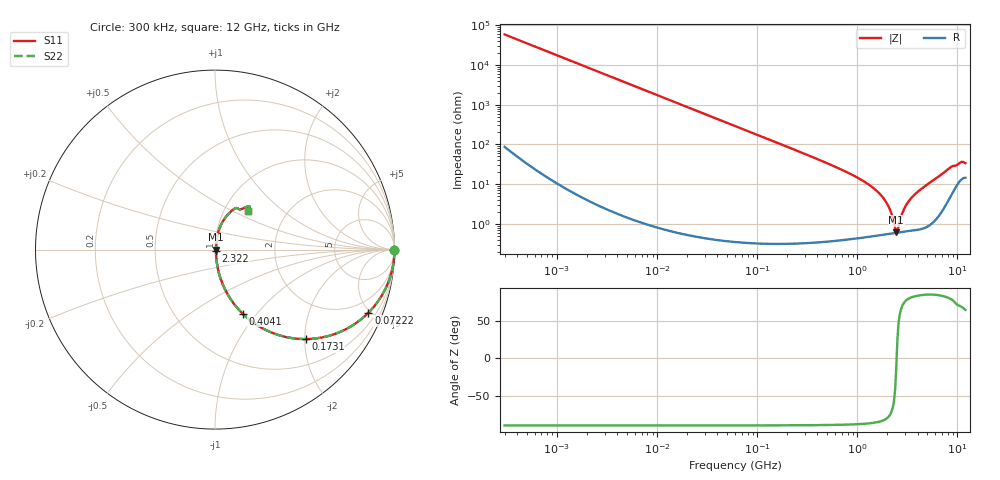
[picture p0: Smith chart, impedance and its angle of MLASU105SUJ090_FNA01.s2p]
! MLASU105SUJ090_FNA01  S-PARAMETER MODEL  ( General Type )
! Model Generated by TAIYO YUDEN Corporation (http://www.ty-top.com)
! Version 2.0
! TAIYO YUDEN Control No. 120810
! Copyright(c) 2012 TAIYO YUDEN CO.,LTD. All Rights Reserved.
! Product Description (link to TY-COMPAS)
! https://ds.yuden.co.jp/TYCOMPAS/or/detail?pn=MLASU105SUJ090DFNA01&u=M
! Products Name : Multilayer Ceramic Capacitors
! Characteristics :
!  Capacitance : 9 pF , Rated Voltage : 50V , TCC : UJ / U2J
!  Case Size : 1.0 x 0.5 / 0.039 x 0.02 [mm/inch] , Thickness : 0.5 / 0.02 [mm/inch]
!  (Conditions: Temperature = 25 degC , DC Bias Current/Voltage = 0A / 0V)
! External Node Assignments :
!  1  o---| |---o  2
! GND o---------o GND
! Frequency Range : 0.3MHz  -  12000MHz  [ 401 STEP ]
# MHz S RI R 50
! Freq[MHz].  S11 Real  S11 Imag  S21 Real  S21 Imag  S12 Real  S12 Imag  S22 Real  S22 Imag
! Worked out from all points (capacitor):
!   401 points, 300 kHz to 12 GHz, reference 50 ohm
!   read as one part in series: C = 9.07 pF near 316.3 kHz
!   lowest |Z| = 612 mohm at 2.448 GHz (marker M1)
!   series resonance near 2.469 GHz, so ESL is about 460 pH
!   S11 on the Smith chart (normalised r, x): 300 kHz: open; 72.22 MHz: 1.01, -4.86; 173.1 MHz: 1.01, -2.02; 404.1 MHz: 1.01, -0.85; 2.322 GHz: 1.01, -0.02; 12 GHz: 1.29, +0.61
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0.3  1 -0.00171  5.46e-06 0.00171  5.46e-06 0.00171  1 -0.00171
1.769972  0.9999 -0.0101  0.000106 0.0101  0.000106 0.0101  0.9999 -0.0101
10.44266  0.9964 -0.0593  0.00356 0.0593  0.00356 0.0593  0.9964 -0.0593
26.39317  0.9778 -0.147  0.0222 0.147  0.0222 0.147  0.9778 -0.147
60  0.895 -0.306  0.105 0.306  0.105 0.306  0.895 -0.306
72.22496  0.8546 -0.3518  0.1454 0.3518  0.1454 0.3518  0.8546 -0.3518
173.124  0.5044 -0.4984  0.4956 0.4984  0.4956 0.4984  0.5044 -0.4984
353.9943  0.1925 -0.3908  0.8075 0.3908  0.8075 0.3908  0.1925 -0.3908
404.1309  0.1536 -0.3565  0.8464 0.3565  0.8464 0.3565  0.1536 -0.3565
783.7017  0.0426 -0.1922  0.9574 0.1922  0.9574 0.1922  0.0426 -0.1922
1262.535  0.015 -0.1009  0.985 0.1009  0.985 0.1009  0.015 -0.1009
1735.023  0.00783 -0.0508  0.9922 0.0508  0.9922 0.0508  0.00783 -0.0508
2088.533  0.00618 -0.024  0.9938 0.024  0.9938 0.024  0.00618 -0.024
2321.999  0.00591 -0.00903  0.9941 0.00903  0.9941 0.00903  0.00591 -0.00903
2448.343  0.00595 -0.00128  0.994 0.00128  0.994 0.00128  0.00595 -0.00128
2581.562  0.00613 0.00654  0.9939 -0.00654  0.9939 -0.00654  0.00613 0.00654
2795.104  0.00656 0.0165  0.9934 -0.0165  0.9934 -0.0165  0.00656 0.0165
3107.553  0.00744 0.0301  0.9926 -0.0301  0.9926 -0.0301  0.00744 0.0301
3841.137  0.0103 0.0572  0.9897 -0.0572  0.9897 -0.0572  0.0103 0.0572
8503.825  0.1016 0.2231  0.8984 -0.2231  0.8984 -0.2231  0.1016 0.2231
10793.46  0.184 0.2417  0.816 -0.2417  0.816 -0.2417  0.184 0.2417
12000  0.1847 0.2175  0.8153 -0.2175  0.8153 -0.2175  0.1847 0.2175
